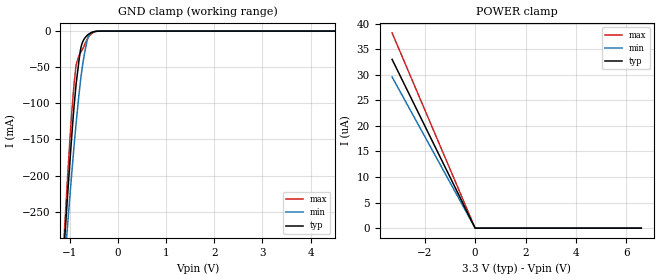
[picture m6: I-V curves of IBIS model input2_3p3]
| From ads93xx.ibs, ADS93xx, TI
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|   input2_3p3 Model
[Model]   input2_3p3
Model_type   Input
Vinl = 0.5
Vinh = 2.8
|   typ   min   max
C_comp   0.610pF   0.583pF   0.633pF
[Voltage Range]   3.3   3   3.5
[Temperature Range]   27   125   -40
[Power Clamp Reference]   3.3   3   3.5
[GND Clamp Reference]   0   0   0
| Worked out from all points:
|   GND clamp passes 1 mA (typ) near -0.51 V on its own axis
[GND Clamp]
|   Voltage   I(typ)   I(min)   I(max)
-3.3V     -2.515A    -2.211A    -2.848A
-1.132V   -307.9mA   -338.1mA   -294.1mA
-1.073V   -248mA     -286.6mA   -225.7mA
-1.063V   -238.2mA   -278.1mA   -214.5mA
-973.5mV  -152.9mA   -203.7mA   -120.3mA
-924mV    -109.8mA   -164.5mA   -78.87mA
-874.5mV  -73.43mA   -127.7mA   -46.75mA
-785.4mV  -26.99mA   -70.3mA    -30.32mA
-706.2mV  -10.95mA   -33.71mA   -20.35mA
-627mV    -4.995mA   -8.749mA   -9.501mA
-537.9mV  -1.596mA   -1.344mA   -2.882mA
6.6V      0A         0A         0A
[POWER Clamp]
|   Voltage   I(typ)   I(min)   I(max)
-3.3V     33uA       29.56uA    38.18uA
-3.3mV    26.22nA    23.75nA    31.18nA
16.5mV    0A         0A         0A
6.6V      0A         0A         0A
